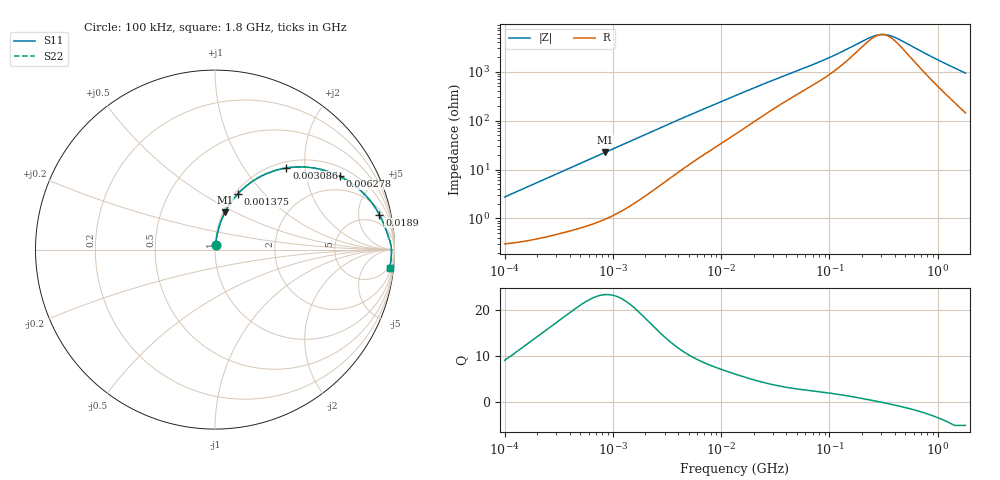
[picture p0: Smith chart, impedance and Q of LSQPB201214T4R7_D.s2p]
! LSQPB201214T4R7_D  S-PARAMETER MODEL  ( General Type )
! Model Generated by TAIYO YUDEN Corporation (http://www.ty-top.com)
! Version 1.0
! TAIYO YUDEN Control No. 100901NG22SB-FKC
! Copyright(c) 2010 TAIYO YUDEN CO.,LTD. All Rights Reserved.
! Product Description (link to TY-COMPAS)
! https://ds.yuden.co.jp/TYCOMPAS/or/detail?pn=LSQPB201214T4R7MD&u=M
! Products Name : Inductors
! Characteristics :
!  Inductance : 4.7 uH , SRF(min) : 250 MHz , DC Resistance(max) : 0.3445 Ohm
!  Rated Current : Saturation :700 mA , Temp Rise : 600 mA (40 degC)
!  Case Size : 2.0 x 1.25 / 0.079 x 0.049 [mm/inch] , Thickness : 1.4 / 0.056 [mm/inch]
!  (Conditions: Temperature = 25 degC , DC Bias Current/Voltage = 0A / 0V)
! External Node Assignments :
!  1  o---GGG---o  2
! GND o---------o GND
! Frequency Range : 0.1MHz  -  1800MHz  [ 402 STEP ]
# MHz S RI R 50
! Freq[MHz].  S11 Real  S11 Imag  S21 Real  S21 Imag  S12 Real  S12 Imag  S22 Real  S22 Imag
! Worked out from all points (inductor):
!   401 points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, 100 kHz to 1.8 GHz, reference 50 ohm
!   read as one part in series: L = 4.33 uH near 105 kHz
!   highest Q = 23.2 at 842.4 kHz (marker M1), where L = 4.21 uH
!   self-resonance near 302.9 MHz
!   S11 on the Smith chart (normalised r, x): 100 kHz: 1.01, +0.05; 1.375 MHz: 1.03, +0.72; 3.086 MHz: 1.12, +1.60; 6.278 MHz: 1.35, +3.14; 18.9 MHz: 2.73, +8.66; 1.8 GHz: 4, -19
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0.1  0.00374 0.0271  0.9963 -0.0271  0.9963 -0.0271  0.00374 0.0271
0.247521  0.00861 0.0659  0.9914 -0.0659  0.9914 -0.0659  0.00861 0.0659
0.516129  0.0246 0.1332  0.9754 -0.1332  0.9754 -0.1332  0.0246 0.1332
0.842407  0.0556 0.2086  0.9444 -0.2086  0.9444 -0.2086  0.0556 0.2086
1.374945  0.1272 0.3107  0.8728 -0.3107  0.8728 -0.3107  0.1272 0.3107
1.890522  0.21 0.3814  0.79 -0.3814  0.79 -0.3814  0.21 0.3814
2.66389  0.3356 0.4405  0.6644 -0.4405  0.6644 -0.4405  0.3356 0.4405
3.085641  0.3982 0.4548  0.6018 -0.4548  0.6018 -0.4548  0.3982 0.4548
4.347904  0.5498 0.4546  0.4502 -0.4546  0.4502 -0.4546  0.5498 0.4546
6.278453  0.6946 0.4085  0.3054 -0.4085  0.3054 -0.4085  0.6946 0.4085
9.066201  0.8027 0.3366  0.1973 -0.3366  0.1973 -0.3366  0.8027 0.3366
13.41641  0.8773 0.2562  0.1227 -0.2562  0.1227 -0.2562  0.8773 0.2562
18.90474  0.9161 0.1948  0.0839 -0.1948  0.0839 -0.1948  0.9161 0.1948
34.03197  0.95 0.1183  0.05 -0.1183  0.05 -0.1183  0.95 0.1183
69.24595  0.9692 0.0634  0.0308 -0.0634  0.0308 -0.0634  0.9692 0.0634
115.8234  0.9773 0.0368  0.0227 -0.0368  0.0227 -0.0368  0.9773 0.0368
247.5026  0.9825 0.00706  0.0175 -0.00706  0.0175 -0.00706  0.9825 0.00706
301.0823  0.9829 0.000203  0.0171 -0.000203  0.0171 -0.000203  0.9829 0.000203
357.3983  0.9832 -0.00583  0.0168 0.00583  0.0168 0.00583  0.9832 -0.00583
434.7684  0.9832 -0.013  0.0168 0.013  0.0168 0.013  0.9832 -0.013
952.0939  0.9812 -0.0498  0.0188 0.0498  0.0188 0.0498  0.9812 -0.0498
1800  0.9733 -0.101  0.0267 0.101  0.0267 0.101  0.9733 -0.101
